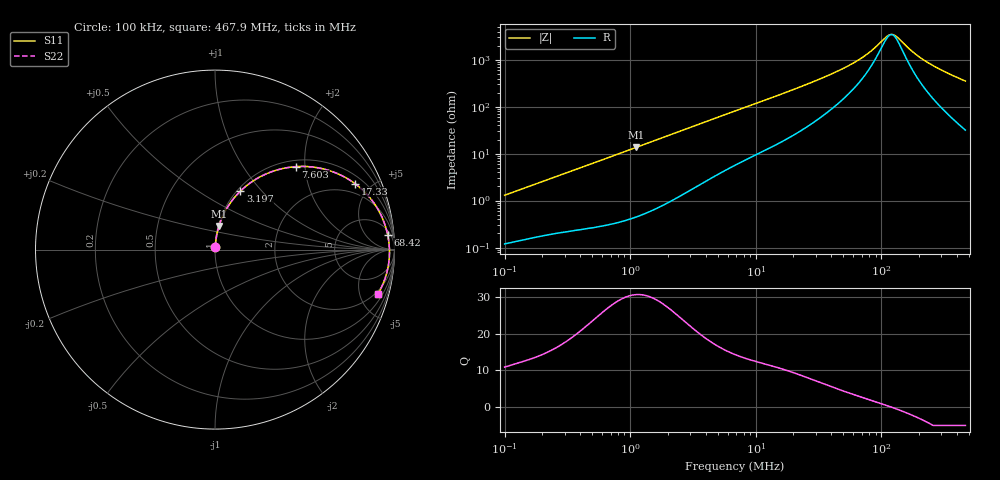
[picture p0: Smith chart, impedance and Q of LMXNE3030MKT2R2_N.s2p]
! LMXNE3030MKT2R2_N  S-PARAMETER MODEL  ( General Type )
! Model Generated by TAIYO YUDEN Corporation (http://www.ty-top.com)
! Version 1.0
! TAIYO YUDEN Control No. 191023NI43SB-FBB
! Copyright(c) 2019 TAIYO YUDEN CO.,LTD. All Rights Reserved.
! Product Description (link to TY-COMPAS)
! https://ds.yuden.co.jp/TYCOMPAS/or/detail?pn=LMXNE3030MKT2R2MN&u=M
! Products Name : Inductors
! Characteristics :
!  Inductance : 2.2 uH , SRF(min) : 78 MHz , DC Resistance(max) : 0.09 Ohm
!  Rated Current : Saturation :1500 mA , Temp Rise : 1370 mA
!  Case Size : 3.0 x 3.0 / 0.118 x 0.118 [mm/inch] , Thickness : 1.2 / 0.047 [mm/inch]
!  (Conditions: Temperature = 25 degC , DC Bias Current/Voltage = 0A / 0V)
! External Node Assignments :
!  1  o---GGG---o  2
! GND o---------o GND
! Frequency Range : 0.1MHz  -  467.920999MHz  [ 402 STEP ]
# MHz S RI R 50
! Freq[MHz].  S11 Real  S11 Imag  S21 Real  S21 Imag  S12 Real  S12 Imag  S22 Real  S22 Imag
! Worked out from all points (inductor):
!   401 points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, 100 kHz to 467.9 MHz, reference 50 ohm
!   read as one part in series: L = 2.04 uH near 104.3 kHz
!   highest Q = 30.6 at 1.112 MHz (marker M1), where L = 1.95 uH
!   self-resonance near 120.2 MHz
!   S11 on the Smith chart (normalised r, x): 100 kHz: 1.00, +0.03; 3.197 MHz: 1.04, +0.77; 7.603 MHz: 1.13, +1.79; 17.33 MHz: 1.40, +4.01; 68.42 MHz: 8, +20; 467.9 MHz: 1.63, -7.03
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0.1  0.00136 0.0129  0.9986 -0.0129  0.9986 -0.0129  0.00136 0.0129
0.411864  0.00499 0.0505  0.995 -0.0505  0.995 -0.0505  0.00499 0.0505
1.11173  0.0223 0.1324  0.9777 -0.1324  0.9777 -0.1324  0.0223 0.1324
1.69632  0.0473 0.1957  0.9527 -0.1957  0.9527 -0.1957  0.0473 0.1957
3.197207  0.1416 0.3259  0.8584 -0.3259  0.8584 -0.3259  0.1416 0.3259
4.676581  0.2515 0.4057  0.7485 -0.4057  0.7485 -0.4057  0.2515 0.4057
6.986533  0.412 0.4581  0.588 -0.4581  0.588 -0.4581  0.412 0.4581
7.602622  0.4494 0.4622  0.5506 -0.4622  0.5506 -0.4622  0.4494 0.4622
11.12042  0.6176 0.446  0.3824 -0.446  0.3824 -0.446  0.6176 0.446
17.33027  0.7801 0.3675  0.2199 -0.3675  0.2199 -0.3675  0.7801 0.3675
28.17346  0.8895 0.2537  0.1105 -0.2537  0.1105 -0.2537  0.8895 0.2537
46.77896  0.9435 0.1477  0.0565 -0.1477  0.0565 -0.1477  0.9435 0.1477
68.42397  0.9619 0.083  0.0381 -0.083  0.0381 -0.083  0.9619 0.083
82.75365  0.9671 0.054  0.0329 -0.054  0.0329 -0.054  0.9671 0.054
106.6332  0.9711 0.0172  0.0289 -0.0172  0.0289 -0.0172  0.9711 0.0172
116.0364  0.9718 0.00511  0.0282 -0.00511  0.0282 -0.00511  0.9718 0.00511
123.629  0.9721 -0.00401  0.0279 0.00401  0.0279 0.00401  0.9721 -0.00401
131.7185  0.9722 -0.0132  0.0278 0.0132  0.0278 0.0132  0.9722 -0.0132
180.8332  0.9698 -0.0609  0.0302 0.0609  0.0302 0.0609  0.9698 -0.0609
237.99  0.9625 -0.1067  0.0375 0.1067  0.0375 0.1067  0.9625 -0.1067
333.7072  0.9435 -0.1721  0.0565 0.1721  0.0565 0.1721  0.9435 -0.1721
467.921  0.9065 -0.2494  0.0935 0.2494  0.0935 0.2494  0.9065 -0.2494
